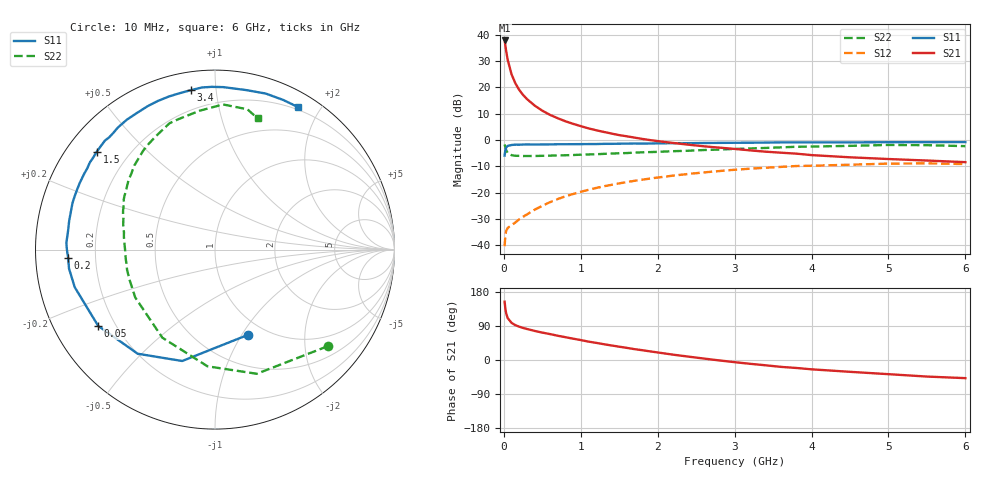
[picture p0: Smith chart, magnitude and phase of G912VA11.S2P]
! SIEMENS Small Signal Semiconductors
! BFG235
! Si NPN RF Bipolar Junction Transistor in SOT223
! VCE = 12 V  IC = 110 mA
! Common Emitter S-Parameters:  July  1994
# GHz  S  MA  R  50
!  f  S11  S21  S12  S22
! GHz  MAG  ANG  MAG  ANG  MAG  ANG  MAG  ANG
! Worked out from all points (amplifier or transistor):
!   40 points, 10 MHz to 6 GHz, reference 50 ohm
!   highest |S21| = 37.9 dB at 10 MHz (marker M1)
!   |S21| within 3 dB of that: start of sweep to 25.39 MHz
!   unconditionally stable (mu >= 1): 479.7 MHz to 1.463 GHz
!   at 200 MHz: K = 0.76, MSG = 24.6 dB, |S12| = -30.1 dB
!   at 1.5 GHz: K = 1.00, MSG = 9.2 dB, |S12| = -16.4 dB
!   at 6 GHz: K = 0.90, MSG = 0.4 dB, |S12| = -9.1 dB
!   S11 on the Smith chart (normalised r, x): 10 MHz: 0.83, -1.06; 50 MHz: 0.14, -0.29; 200 MHz: 0.10, -0.03; 1.5 GHz: 0.09, +0.36; 3.4 GHz: 0.09, +0.86; 6 GHz: 0.17, +1.73
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0.01  0.5093 -69.1  78.11 153.8  0.0097 64.0  0.8272 -40.6
0.02  0.647 -106.4  62.61 135.4  0.0156 49.5  0.7299 -71.4
0.03  0.7226 -126.6  49.72 123.5  0.0188 42.5  0.6516 -93.7
0.05  0.7773 -146.9  33.5 110.6  0.0215 33.1  0.5716 -120.9
0.1  0.8092 -165.0  17.81 98.0  0.0244 33.8  0.5183 -149.0
0.15  0.8202 -172.6  11.98 91.9  0.0274 39.6  0.5049 -160.6
0.2  0.8195 -176.7  8.969 87.9  0.0314 44.1  0.5028 -167.0
0.25  0.8253 179.9  7.223 84.6  0.035 47.7  0.4996 -171.2
0.3  0.829 177.4  6.037 81.9  0.0388 51.1  0.5 -174.6
0.4  0.8253 172.5  4.539 76.8  0.0477 55.2  0.5002 -179.0
0.5  0.8282 168.8  3.623 72.3  0.0567 57.2  0.5039 177.5
0.6  0.83 165.6  3.02 68.4  0.0664 58.2  0.5081 174.4
0.7  0.8355 161.8  2.608 64.0  0.076 58.5  0.5131 171.7
0.9  0.838 156.4  2.04 56.3  0.0948 57.2  0.5219 167.2
1.1  0.8424 150.0  1.672 48.5  0.1139 55.2  0.5352 162.7
1.5  0.8556 140.3  1.246 35.1  0.151 49.4  0.5634 154.7
2.2  0.8747 124.2  0.885 14.1  0.2117 37.3  0.6168 141.5
3.2  0.8934 102.7  0.639 -10.0  0.287 18.1  0.6946 122.3
3.4  0.8985 98.5  0.604 -13.9  0.2988 14.0  0.7111 117.9
4.5  0.9056 78.9  0.472 -31.2  0.3415 -7.1  0.7788 96.2
5.5  0.9163 65.5  0.41 -43.7  0.3623 -25.7  0.8023 77.0
6  0.919 59.7  0.382 -47.9  0.3517 -32.7  0.7689 72.0
